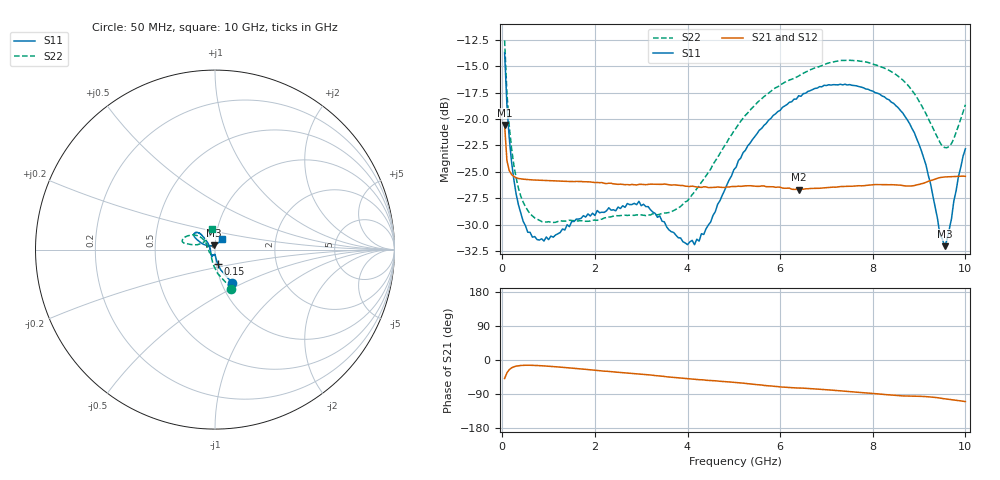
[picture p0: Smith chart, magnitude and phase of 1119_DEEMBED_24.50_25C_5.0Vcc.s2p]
!Hittite Microwave Corp.
!Digital Attenuator/PhaseShifter Rev 1.4.0
!Filename: C:\DATA\DATA\1119_DEEMBED_24.50_25C_5.0Vcc.s2p
!VNA ID: Agilent Technologies,N5224A,MY51441122,A.10.45.03
!Device type:
!2 Port Calibration.
!Temp(C): 25
!Lot Number:
!Serial Number:
!Operator:
!Misc:
!Attenuator:  24.500
# GHZ S DB R 50.0
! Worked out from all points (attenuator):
!   200 points, 50 MHz to 10 GHz, reference 50 ohm
!   highest |S21| = -20.55 dB at 50 MHz (marker M1); lowest = -26.7 dB at 6.4 GHz (marker M2)
!   lowest |S11| = -32.0 dB at 9.55 GHz (marker M3), VSWR 1.05, Z = 49.3 + j2.39 ohm
!   |S11| at or under -10 dB: start of sweep to end of sweep
!   |S22| runs from -29.8 to -12.6 dB; largest |S21 - S12| = 0.00014
!   S11 on the Smith chart (normalised r, x): 50 MHz: 1.12, -0.43; 150 MHz: 1.02, -0.16; 10 GHz: 1.07, +0.13
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0.05  -13.69 -62.9  -20.55 -48.7  -20.55 -48.7  -12.55 -67.2
0.1  -18.68 -74.5  -23.93 -34.0  -23.93 -34.0  -17.51 -83.9
0.15  -21.79 -79.2  -24.89 -25.5  -24.89 -25.4  -20.64 -93.4
0.25  -25.75 -82.8  -25.45 -17.9  -25.46 -17.9  -24.37 -105.9
0.35  -28.15 -84.8  -25.63 -15.2  -25.62 -15.1  -26.58 -114.5
0.65  -31.20 -90.9  -25.77 -14.0  -25.77 -14.1  -29.18 -130.0
1  -31.43 -97.0  -25.84 -16.4  -25.85 -16.4  -29.73 -137.0
1.75  -29.16 -110.4  -25.94 -24.1  -25.94 -24.1  -29.65 -140.6
2.95  -27.80 -118.2  -26.19 -36.7  -26.20 -36.8  -29.10 -159.8
3.4  -29.18 -131.7  -26.19 -42.0  -26.19 -42.1  -29.02 -173.3
4.15  -31.91 -177.9  -26.40 -51.1  -26.40 -51.2  -26.92 156.2
4.5  -29.76 155.7  -26.49 -54.2  -26.51 -54.2  -24.74 145.1
5.05  -24.56 135.9  -26.39 -59.4  -26.41 -59.5  -20.83 138.9
5.55  -21.06 132.2  -26.38 -65.5  -26.39 -65.5  -18.26 141.3
6.4  -17.79 133.9  -26.69 -73.9  -26.70 -73.9  -15.92 150.0
6.7  -17.20 136.7  -26.57 -76.1  -26.58 -76.1  -15.24 154.0
7.5  -16.73 144.4  -26.37 -83.4  -26.37 -83.4  -14.43 163.6
8.35  -18.17 149.8  -26.23 -91.9  -26.23 -91.9  -15.38 168.1
8.999999  -22.41 155.1  -26.20 -95.8  -26.20 -95.8  -18.31 167.3
9.55  -32.05 104.6  -25.49 -102.3  -25.50 -102.3  -22.70 138.1
9.7  -29.45 71.1  -25.46 -104.7  -25.47 -104.7  -22.32 119.9
10  -22.82 57.3  -25.43 -109.7  -25.43 -109.7  -18.64 98.5
